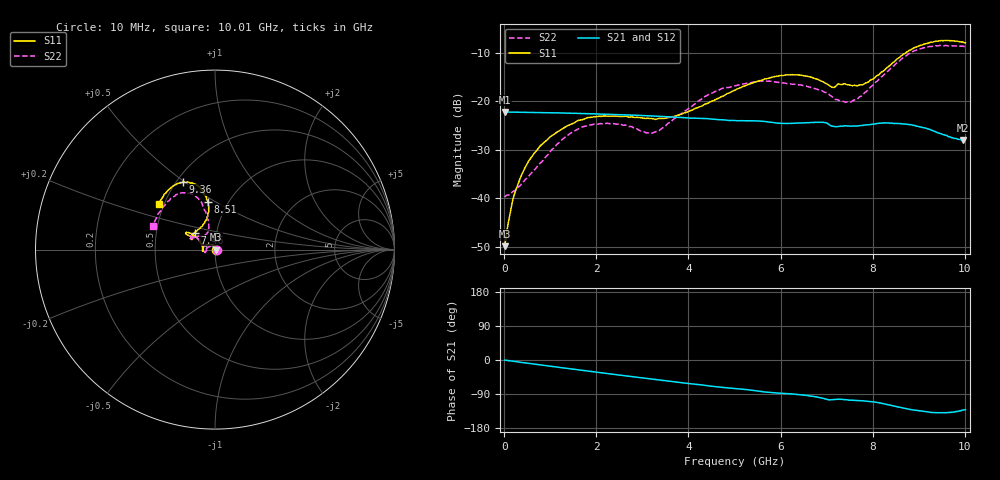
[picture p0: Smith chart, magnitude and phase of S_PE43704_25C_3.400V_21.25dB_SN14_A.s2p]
! Device ID: PE43704
! Dir: z:\PE43704\PE43704_Char_1_20130516\PE43704\AMB\3p400V\21p25dB
! Serial: 14
! Insertion: A
! Impedance: 50 ohm
! Temp: Amb
! VDD: 3.400V
! Attenuation Step: 21.25dB
! IDD: 1.140292e-01mA
#  Hz  S  RI  R  50
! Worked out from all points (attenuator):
!   401 points, 10 MHz to 10.01 GHz, reference 50 ohm
!   highest |S21| = -22.21 dB at 10 MHz (marker M1); lowest = -28.0 dB at 9.96 GHz (marker M2)
!   lowest |S11| = -49.9 dB at 10 MHz (marker M3), VSWR 1.01, Z = 50.3 + j0.0502 ohm
!   |S11| at or under -10 dB: start of sweep to 8.718 GHz
!   |S22| runs from -39.7 to -8.5 dB; largest |S21 - S12| = 0.00079
!   S11 on the Smith chart (normalised r, x): 10 MHz: 1.01, +0.00; 7.46 GHz: 0.78, +0.15; 8.51 GHz: 0.81, +0.46; 9.36 GHz: 0.54, +0.49; 10.01 GHz: 0.47, +0.28
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1e7  0.00316 0.000499  0.0776 -0.000245  0.0775 -0.000249  0.0103 0.000288
1.6e8  0.00278 0.00789  0.0773 -0.00373  0.0773 -0.0037  0.00971 0.00593
2.35e8  0.00135 0.0114  0.0771 -0.00538  0.0771 -0.00533  0.00826 0.00871
5.35e8  -0.0072 0.0232  0.076 -0.0118  0.076 -0.0118  -0.000634 0.0169
1.035e9  -0.0326 0.0299  0.0729 -0.0221  0.0729 -0.0221  -0.026 0.0182
1.685e9  -0.0625 0.0156  0.0665 -0.0342  0.0666 -0.0342  -0.0542 -0.00108
2.26e9  -0.07 -0.00157  0.0592 -0.0432  0.0593 -0.0432  -0.0572 -0.0152
3.11e9  -0.0666 -0.00606  0.0465 -0.0536  0.0465 -0.0536  -0.0471 -0.00176
3.36e9  -0.0666 -0.00022  0.0421 -0.0558  0.0422 -0.0557  -0.0491 0.0082
4.41e9  -0.0842 0.0442  0.025 -0.0613  0.0251 -0.0613  -0.0968 0.0623
5.01e9  -0.108 0.0726  0.0162 -0.0612  0.0162 -0.0613  -0.1261 0.0709
5.96e9  -0.1557 0.0962  0.00285 -0.0595  0.00305 -0.0595  -0.1403 0.0692
6.685e9  -0.1556 0.0827  -0.00613 -0.0603  -0.00618 -0.0604  -0.1217 0.0652
7.11e9  -0.1249 0.0644  -0.0141 -0.0538  -0.0143 -0.0538  -0.0832 0.0752
7.46e9  -0.114 0.0943  -0.0147 -0.0537  -0.0149 -0.0538  -0.0521 0.0845
7.835e9  -0.0675 0.138  -0.0181 -0.054  -0.0178 -0.0537  -0.035 0.119
8.36e9  -0.0352 0.2296  -0.0286 -0.0523  -0.0288 -0.0524  -0.0503 0.2054
8.51e9  -0.038 0.265  -0.0321 -0.0496  -0.0319 -0.0499  -0.063 0.2381
8.935e9  -0.089 0.3504  -0.0379 -0.0409  -0.0381 -0.0408  -0.1301 0.3091
9.36e9  -0.1786 0.3763  -0.0367 -0.0319  -0.0367 -0.0314  -0.2185 0.3049
9.96e9  -0.3051 0.271  -0.0267 -0.0297  -0.0269 -0.0297  -0.3386 0.151
1.001e10  -0.3128 0.2515  -0.0263 -0.0302  -0.0265 -0.0302  -0.3444 0.1303
